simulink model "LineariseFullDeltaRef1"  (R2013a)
settings: Solver=ode23tb  StartTime=0.0  StopTime=2  RelTol=1e-3
InitFcn:
  | SimParam.IC = SM2_InitCondConstrFnc(RawParam,IC);
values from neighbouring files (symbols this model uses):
  RawParam = RobotParamGather(ParamLib)    [main_testIdentification3quad.m]    (also in main_testIdentification_fullRobot.m; main_testIdentification_fullRobot1.m; DeltaModelMain_v2.m; main_TimeSimulation.m)
libraries: SM2_ArmPartsLib x12, SM2_BallJointPartsLib x6, SM2_ForeArmPartsLib x6, SM2_MotorPartsLib x3, SM2_FramePartsLib x1, SM2_ToolPartsLib x1

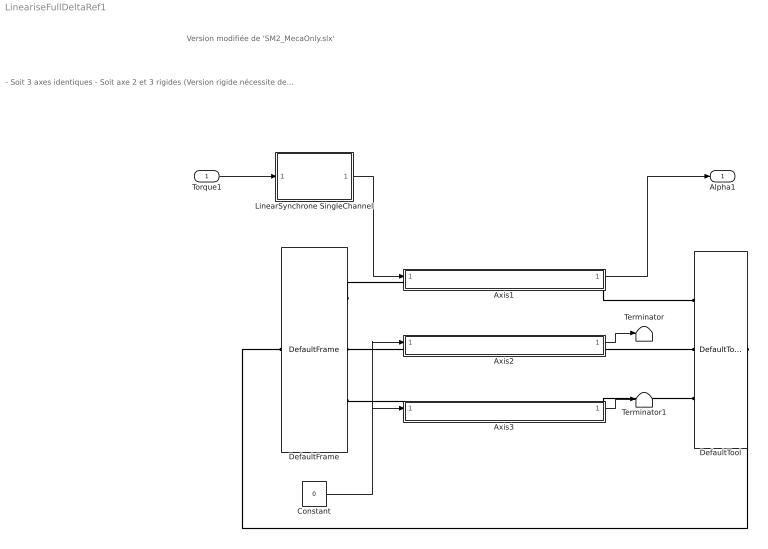
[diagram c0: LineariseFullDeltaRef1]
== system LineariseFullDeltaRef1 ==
  note: - Soit 3 axes identiques - Soit axe 2 et 3 rigides (Version rigide nécessite des blocks non liés au libraries et des fonctions d'initialisaions indépendantes voir "local###_paramInitFnc()")
  note: Version modifiée de 'SM2_MecaOnly.slx'
  Torque1 : Inport
  Axis1 : Subsystem
  Axis2 : Subsystem
  Axis3 : Subsystem
  Constant : Constant  Value=0
  DefaultFrame : SM2_FramePartsLib/DefaultFrame
  DefaultTool : SM2_ToolPartsLib/DefaultTool
  LinearSynchrone SingleChannel : Subsystem  InitFcn=SimParam.Driver = driver_ParamInitFnc(RawParam,2);  VariantControl=driverVarLinearSynchrone
  Terminator : Terminator
  Terminator1 : Terminator
  Alpha1 : Outport
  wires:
  Axis1/1(Alpha) -> Alpha1/1
  LinearSynchrone SingleChannel/1(Torque) -> Axis1/1(Torque)
  Torque1/1 -> LinearSynchrone SingleChannel/1(U)
  Axis3/1(Alpha) -> Terminator1/1
  Axis2/1(Alpha) -> Terminator/1
  Constant/1 -> Axis3/1(Torque), Axis2/1(Torque)
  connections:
  DefaultFrame/RConn1 -- Axis1/LConn1
  Axis1/RConn1 -- DefaultTool/RConn1
  DefaultTool/LConn1 -- DefaultFrame/LConn1
  Axis2/LConn1 -- DefaultFrame/RConn2
  Axis2/RConn1 -- DefaultTool/RConn2
  Axis3/LConn1 -- DefaultFrame/RConn3
  Axis3/RConn1 -- DefaultTool/RConn3

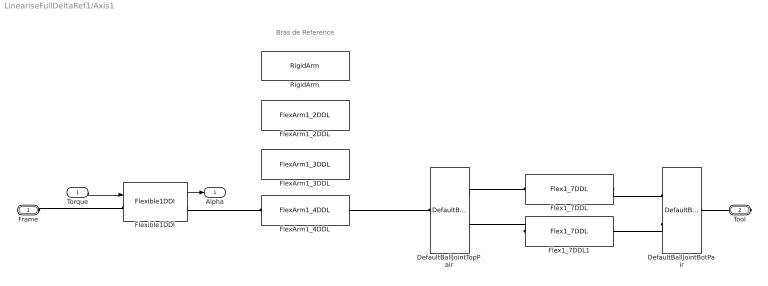
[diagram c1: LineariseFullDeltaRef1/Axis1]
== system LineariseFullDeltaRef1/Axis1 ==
  note: Bras de Reference
  Torque : Inport
  DefaultBallJointBotPair : SM2_BallJointPartsLib/DefaultBallJointBotPair
  DefaultBallJointTopPair : SM2_BallJointPartsLib/DefaultBallJointTopPair
  Flex1_7DDL : SM2_ForeArmPartsLib/Flex1_7DDL  VariantControl=foreArmVarFlex1_7ddl
  Flex1_7DDL1 : SM2_ForeArmPartsLib/Flex1_7DDL  VariantControl=foreArmVarFlex1_7ddl
  FlexArm1_2DDL : SM2_ArmPartsLib/FlexArm1_2DDL  Commented=on  VariantControl=armVarFlex1_2ddl
  FlexArm1_3DDL : SM2_ArmPartsLib/FlexArm1_3DDL  Commented=on  VariantControl=armVarFlex1_3ddl
  FlexArm1_4DDL : SM2_ArmPartsLib/FlexArm1_4DDL  VariantControl=armVarFlex1_4ddl
  Flexible1DDl : SM2_MotorPartsLib/Flexible1DDl  VariantControl=motorVarFlex1
  RigidArm : SM2_ArmPartsLib/RigidArm  Commented=on  VariantControl=armVarDefault
  Frame : PMIOPort  Port=1  Side=Left
  Tool : PMIOPort  Port=2  Side=Right
  Alpha : Outport
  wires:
  Torque/1 -> Flexible1DDl/1
  Flexible1DDl/1 -> Alpha/1
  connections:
  Frame/RConn1 -- Flexible1DDl/LConn1
  Flexible1DDl/RConn1 -- FlexArm1_4DDL/LConn1
  DefaultBallJointTopPair/RConn1 -- FlexArm1_4DDL/RConn1
  Flex1_7DDL1/LConn1 -- DefaultBallJointTopPair/LConn2
  DefaultBallJointTopPair/LConn1 -- Flex1_7DDL/LConn1
  Flex1_7DDL/RConn1 -- DefaultBallJointBotPair/LConn1
  DefaultBallJointBotPair/LConn2 -- Flex1_7DDL1/RConn1
  Tool/RConn1 -- DefaultBallJointBotPair/RConn1

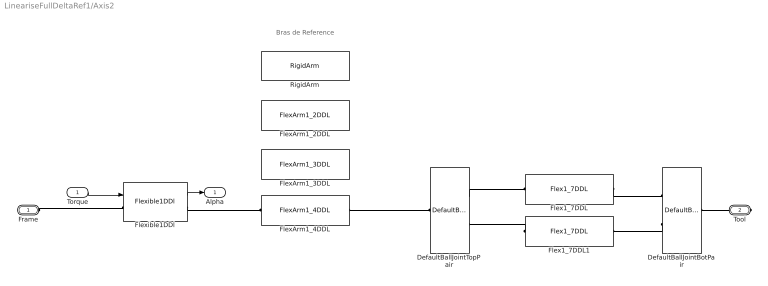
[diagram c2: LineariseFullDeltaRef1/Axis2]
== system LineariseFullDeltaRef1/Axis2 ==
  note: Bras de Reference
  Torque : Inport
  DefaultBallJointBotPair : SM2_BallJointPartsLib/DefaultBallJointBotPair
  DefaultBallJointTopPair : SM2_BallJointPartsLib/DefaultBallJointTopPair
  Flex1_7DDL : SM2_ForeArmPartsLib/Flex1_7DDL  VariantControl=foreArmVarFlex1_7ddl
  Flex1_7DDL1 : SM2_ForeArmPartsLib/Flex1_7DDL  VariantControl=foreArmVarFlex1_7ddl
  FlexArm1_2DDL : SM2_ArmPartsLib/FlexArm1_2DDL  Commented=on  VariantControl=armVarFlex1_2ddl
  FlexArm1_3DDL : SM2_ArmPartsLib/FlexArm1_3DDL  Commented=on  VariantControl=armVarFlex1_3ddl
  FlexArm1_4DDL : SM2_ArmPartsLib/FlexArm1_4DDL  VariantControl=armVarFlex1_4ddl
  Flexible1DDl : SM2_MotorPartsLib/Flexible1DDl  VariantControl=motorVarFlex1
  RigidArm : SM2_ArmPartsLib/RigidArm  Commented=on  VariantControl=armVarDefault
  Frame : PMIOPort  Port=1  Side=Left
  Tool : PMIOPort  Port=2  Side=Right
  Alpha : Outport
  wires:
  Torque/1 -> Flexible1DDl/1
  Flexible1DDl/1 -> Alpha/1
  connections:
  Frame/RConn1 -- Flexible1DDl/LConn1
  Flexible1DDl/RConn1 -- FlexArm1_4DDL/LConn1
  DefaultBallJointTopPair/RConn1 -- FlexArm1_4DDL/RConn1
  Flex1_7DDL1/LConn1 -- DefaultBallJointTopPair/LConn2
  DefaultBallJointTopPair/LConn1 -- Flex1_7DDL/LConn1
  Flex1_7DDL/RConn1 -- DefaultBallJointBotPair/LConn1
  DefaultBallJointBotPair/LConn2 -- Flex1_7DDL1/RConn1
  Tool/RConn1 -- DefaultBallJointBotPair/RConn1

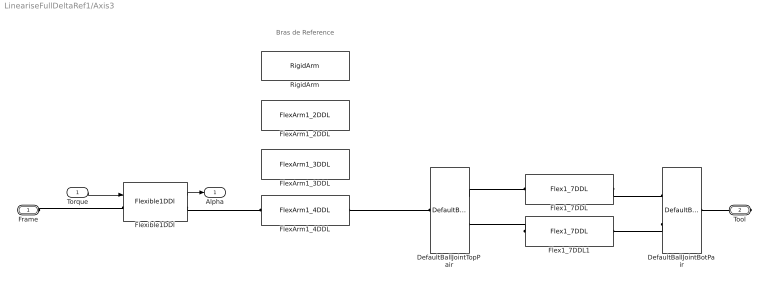
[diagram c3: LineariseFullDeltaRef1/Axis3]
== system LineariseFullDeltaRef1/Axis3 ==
  note: Bras de Reference
  Torque : Inport
  DefaultBallJointBotPair : SM2_BallJointPartsLib/DefaultBallJointBotPair
  DefaultBallJointTopPair : SM2_BallJointPartsLib/DefaultBallJointTopPair
  Flex1_7DDL : SM2_ForeArmPartsLib/Flex1_7DDL  VariantControl=foreArmVarFlex1_7ddl
  Flex1_7DDL1 : SM2_ForeArmPartsLib/Flex1_7DDL  VariantControl=foreArmVarFlex1_7ddl
  FlexArm1_2DDL : SM2_ArmPartsLib/FlexArm1_2DDL  Commented=on  VariantControl=armVarFlex1_2ddl
  FlexArm1_3DDL : SM2_ArmPartsLib/FlexArm1_3DDL  Commented=on  VariantControl=armVarFlex1_3ddl
  FlexArm1_4DDL : SM2_ArmPartsLib/FlexArm1_4DDL  VariantControl=armVarFlex1_4ddl
  Flexible1DDl : SM2_MotorPartsLib/Flexible1DDl  VariantControl=motorVarFlex1
  RigidArm : SM2_ArmPartsLib/RigidArm  Commented=on  VariantControl=armVarDefault
  Frame : PMIOPort  Port=1  Side=Left
  Tool : PMIOPort  Port=2  Side=Right
  Alpha : Outport
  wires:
  Torque/1 -> Flexible1DDl/1
  Flexible1DDl/1 -> Alpha/1
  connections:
  Frame/RConn1 -- Flexible1DDl/LConn1
  Flexible1DDl/RConn1 -- FlexArm1_4DDL/LConn1
  DefaultBallJointTopPair/RConn1 -- FlexArm1_4DDL/RConn1
  Flex1_7DDL1/LConn1 -- DefaultBallJointTopPair/LConn2
  DefaultBallJointTopPair/LConn1 -- Flex1_7DDL/LConn1
  Flex1_7DDL/RConn1 -- DefaultBallJointBotPair/LConn1
  DefaultBallJointBotPair/LConn2 -- Flex1_7DDL1/RConn1
  Tool/RConn1 -- DefaultBallJointBotPair/RConn1

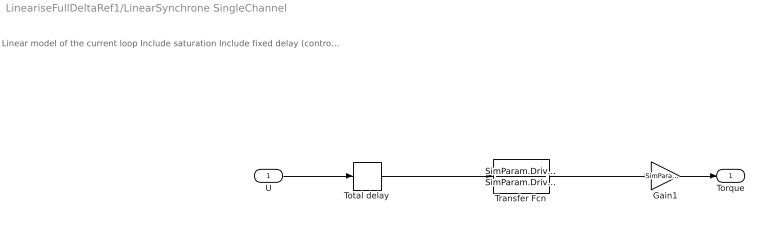
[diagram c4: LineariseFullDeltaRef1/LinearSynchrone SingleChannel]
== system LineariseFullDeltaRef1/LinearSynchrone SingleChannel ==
  note: Linear model of the current loop Include saturation Include fixed delay (control delay + driver delay + 0.5*driver sample periode if assynchonous)
  U : Inport
  Gain1 : Gain  Gain=SimParam.Driver.GRelScale
  Total delay : TransportDelay  DelayTime=SimParam.Driver.tau  BufferSize=10000
  Transfer Fcn : TransferFcn  Numerator=SimParam.Driver.TfNum  Denominator=SimParam.Driver.TfDen
  Torque : Outport
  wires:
  Total delay/1 -> Transfer Fcn/1
  Gain1/1 -> Torque/1
  U/1 -> Total delay/1
  Transfer Fcn/1 -> Gain1/1
